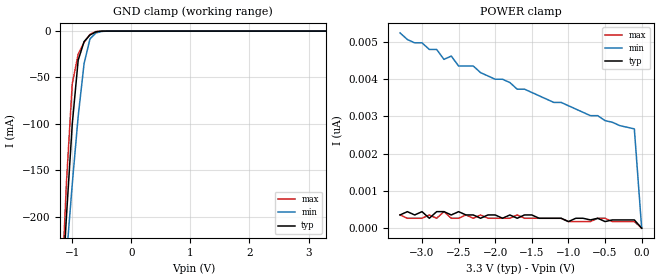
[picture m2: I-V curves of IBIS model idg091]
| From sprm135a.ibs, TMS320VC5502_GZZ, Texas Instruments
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[Model]   idg091
Model_type   Input
Polarity   Non-Inverting
| signals   A, Y
Vinl = 0.8V
Vinh = 2.0V
|   typ   min   max
C_comp   1.5639p   1.4731p   1.7754p
|   typ   min   max
[Temperature Range]   25   -40   125
|   typ   min   max
[Voltage Range]   3.30V   3.00V   3.60V
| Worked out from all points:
|   GND clamp passes 1 mA (typ) near -0.61 V on its own axis
[GND_clamp]
|   Voltage   I(typ)   I(min)   I(max)
-3.3V     -2.941A    -2.221A    -3.818A
-1.2V     -314mA     -328mA     -309.9mA
-1.1V     -201.4mA   -244.7mA   -165mA
-1V       -100.1mA   -164.9mA   -56.77mA
-900mV    -31.41mA   -92.01mA   -24.84mA
-800mV    -11.37mA   -35mA      -12.04mA
-700mV    -4.182mA   -8.432mA   -3.555mA
-600mV    -818.6uA   -2.03mA    -409.7uA
-500mV    -75.21uA   -364.5uA   -19.35uA
-400mV    -4.217uA   -44.76uA   -434.5nA
3.3V      177.6pA    2.753nA    133.2pA
[POWER_clamp]
|   Voltage   I(typ)   I(min)   I(max)
-3.3V     355.3pA    5.24nA     355.3pA
-3V       444.1pA    4.974nA    266.4pA
-2.9V     266.4pA    4.796nA    355.3pA
-2.8V     444.1pA    4.796nA    266.4pA
-2.7V     444.1pA    4.53nA     444.1pA
-2.6V     355.3pA    4.619nA    266.4pA
-2.5V     444.1pA    4.352nA    266.4pA
-2.3V     355.3pA    4.352nA    266.4pA
-2.2V     266.4pA    4.174nA    355.3pA
-1.5V     355.3pA    3.641nA    266.4pA
-100mV    222pA      2.665nA    177.6pA
0V        1pA        1pA        1pA
